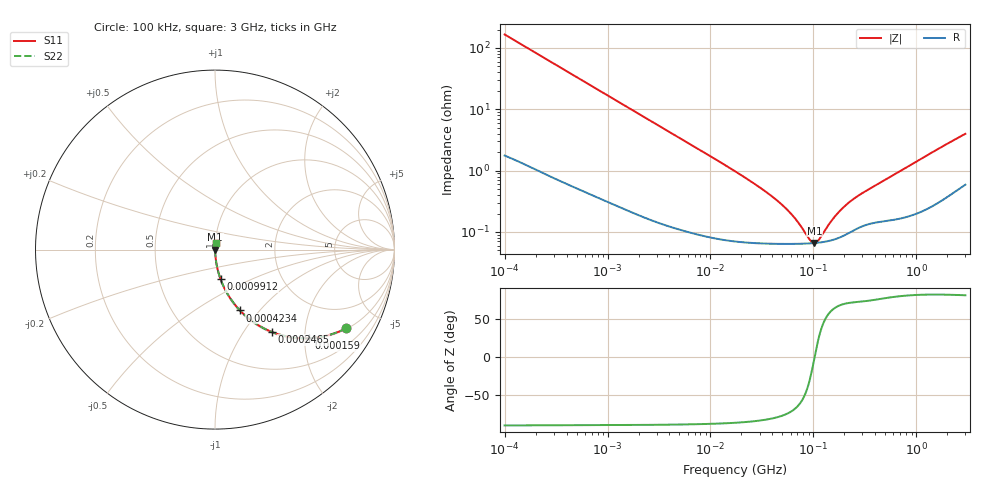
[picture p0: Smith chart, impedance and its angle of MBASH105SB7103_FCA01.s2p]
! MBASH105SB7103_FCA01  S-PARAMETER MODEL  ( Standard Model )
! Model Generated by TAIYO YUDEN Corporation (http://www.ty-top.com)
! Version 1.0
! TAIYO YUDEN Control No. 220601
! Copyright(c) 2019 TAIYO YUDEN CO.,LTD. All Rights Reserved.
! Product Description (link to TY-COMPAS)
! https://ds.yuden.co.jp/TYCOMPAS/or/detail?pn=MBASH105SB7103KFCA01&u=M
! Products Name : Multilayer Ceramic Capacitors
! Characteristics :
!  Capacitance : 0.01 [uF] , Rated Voltage : 100 [V] , TCC : X7R
!  Case Size : 1.0 x 0.5 / 0.039 x 0.02 [mm/inch] , Thickness : 0.5 / 0.02 [mm/inch]
!  (Conditions: Temperature = 25 [degC] , DC Bias Voltage = 0 [V])
! External Node Assignments :
!  1  o---| |---o  2
! GND o---------o GND
! Frequency Range : 100kHz  -  3GHz  [ 401 STEP ]
# MHZ S RI R 50
! Freq[MHz].  S11 Real  S11 Imag  S21 Real  S21 Imag  S12 Real  S12 Imag  S22 Real  S22 Imag
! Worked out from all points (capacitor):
!   401 points, 100 kHz to 3 GHz, reference 50 ohm
!   read as one part in series: C = 9.57 nF near 105.3 kHz
!   lowest |Z| = 66 mohm at 102.5 MHz (marker M1)
!   series resonance near 102.7 MHz, so ESL is about 250 pH
!   S11 on the Smith chart (normalised r, x): 100 kHz: 1.04, -3.32; 159 kHz: 1.02, -2.09; 246.5 kHz: 1.02, -1.36; 423.4 kHz: 1.01, -0.79; 991.2 kHz: 1.01, -0.34; 3 GHz: 1.01, +0.08
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0.1  0.7315 -0.4379  0.2685 0.4379  0.2685 0.4379  0.7315 -0.4379
0.159027  0.5229 -0.4935  0.4771 0.4935  0.4771 0.4935  0.5229 -0.4935
0.246461  0.3173 -0.459  0.6827 0.459  0.6827 0.459  0.3173 -0.459
0.327242  0.2109 -0.4011  0.7891 0.4011  0.7891 0.4011  0.2109 -0.4011
0.423445  0.1395 -0.3392  0.8605 0.3392  0.8605 0.3392  0.1395 -0.3392
0.562235  0.0858 -0.2724  0.9142 0.2724  0.9142 0.2724  0.0858 -0.2724
0.991196  0.0312 -0.1649  0.9688 0.1649  0.9688 0.1649  0.0312 -0.1649
1.702975  0.0119 -0.0985  0.9881 0.0985  0.9881 0.0985  0.0119 -0.0985
3.161081  0.0043 -0.0538  0.9957 0.0538  0.9957 0.0538  0.0043 -0.0538
17.7727  0.000785 -0.00948  0.9992 0.00948  0.9992 0.00948  0.000785 -0.00948
32.98988  0.00067 -0.00473  0.9993 0.00473  0.9993 0.00473  0.00067 -0.00473
51.12795  0.000645 -0.00257  0.9994 0.00257  0.9994 0.00257  0.000645 -0.00257
66.15861  0.000641 -0.00155  0.9994 0.00155  0.9994 0.00155  0.000641 -0.00155
90.13636  0.00065 -0.000448  0.9994 0.000448  0.9994 0.000448  0.00065 -0.000448
97.38194  0.000655 -0.000183  0.9993 0.000183  0.9993 0.000183  0.000655 -0.000183
102.5331  0.000659 -6.22e-06  0.9993 6.22e-06  0.9993 6.22e-06  0.000659 -6.22e-06
113.6672  0.000671 0.000348  0.9993 -0.000348  0.9993 -0.000348  0.000671 0.000348
154.8634  0.000744 0.00145  0.9993 -0.00145  0.9993 -0.00145  0.000744 0.00145
210.9903  0.000928 0.00266  0.9991 -0.00266  0.9991 -0.00266  0.000928 0.00266
287.4592  0.00122 0.00394  0.9988 -0.00394  0.9988 -0.00394  0.00122 0.00394
547.5153  0.00159 0.00756  0.9984 -0.00756  0.9984 -0.00756  0.00159 0.00756
3000  0.0074 0.0389  0.9926 -0.0389  0.9926 -0.0389  0.0074 0.0389
